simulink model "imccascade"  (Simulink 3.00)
settings: Solver=ode45  SolverMode=SingleTasking  StartTime=0.0  StopTime=100  FixedStep=st_size  MaxStep=st_size  RelTol=1e-5  AbsTol=1e-6
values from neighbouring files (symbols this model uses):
  Disturb = Setpoint    [mimo_MSF1DF_sim.m]    (also in mimo_MSF2DF_sim.m)
  Satlb = temp1    [cback.m]    (also in imcmenu.m = str2num(satlbs))
  Satub = temp1    [cback.m]    (also in imcmenu.m = str2num(satubs))
  Setpoint = zeros(1,n)    [mimo_MSF1DF_sim.m]    (also in mimo_MSF2DF_sim.m)
undefined symbols (not defined in the file or in its folder): denCs, denCs2, numCs, numCs2, Qdden, Qdnum, XdenMs, XdenPs, Xmdeadx, XnumMs, XnumPs, Xpdeadx

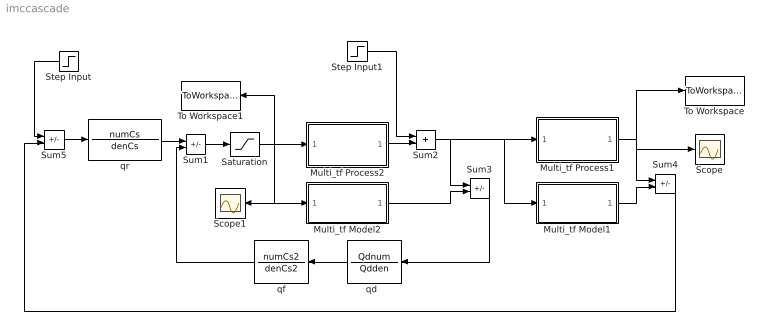
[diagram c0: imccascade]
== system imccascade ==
  Multi_tf Model1 : Subsystem
  Multi_tf Model2 : Subsystem
  Multi_tf Process1 : Subsystem
  Multi_tf Process2 : Subsystem
  Saturation : Saturate  UpperLimit=Satub  LowerLimit=Satlb
  Scope : Scope
  Scope1 : Scope
  Step Input : Step  Orientation=left  Time=0  Before=0  After=Setpoint  SampleTime=0
  Step Input1 : Step  Time=0  Before=0  After=Disturb  SampleTime=0
  Sum{1,3..5} (4 alike) : Sum  Inputs=+-  SaturateOnIntegerOverflow=on
  Sum2 : Sum  Inputs=++  SaturateOnIntegerOverflow=on
  To Workspace : ToWorkspace  VariableName=simout  SampleTime=-1  SaveFormat=Matrix
  To Workspace1 : ToWorkspace  VariableName=effort  SampleTime=-1  SaveFormat=Matrix
  "qd  " : TransferFcn  Orientation=left  Numerator=Qdnum  Denominator=Qdden
  qf : TransferFcn  Orientation=left  Numerator=numCs2  Denominator=denCs2
  qr : TransferFcn  Numerator=numCs  Denominator=denCs
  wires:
  qr/1 -> Sum1/1
  Sum3/1 -> "qd  "/1
  "qd  "/1 -> qf/1
  qf/1 -> Sum1/2
  Sum1/1 -> Saturation/1
  Multi_tf Model2/1(Out1) -> Sum3/2
  Saturation/1 -> Multi_tf Process2/1(In1), Multi_tf Model2/1(In1), Scope1/1, To Workspace1/1
  Multi_tf Process2/1(Out1) -> Sum2/2
  Step Input1/1 -> Sum2/1
  Sum2/1 -> Sum3/1, Multi_tf Process1/1(In1), Multi_tf Model1/1(In1)
  Multi_tf Model1/1(Out1) -> Sum4/2
  Multi_tf Process1/1(Out1) -> To Workspace/1, Sum4/1, Scope/1
  Sum4/1 -> Sum5/2
  Sum5/1 -> qr/1
  Step Input/1 -> Sum5/1

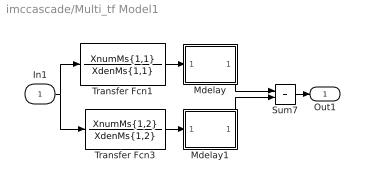
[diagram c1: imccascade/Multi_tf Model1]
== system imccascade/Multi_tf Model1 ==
  In1 : Inport  Port=1  PortWidth=-1  SampleTime=-1  DataType=auto
  Mdelay : Subsystem
  Mdelay1 : Subsystem
  Sum7 : Sum  Inputs=++  SaturateOnIntegerOverflow=on
  Transfer Fcn1 : TransferFcn  Numerator=XnumMs{1,1}  Denominator=XdenMs{1,1}
  Transfer Fcn3 : TransferFcn  Numerator=XnumMs{1,2}  Denominator=XdenMs{1,2}
  Out1 : Outport  Port=1  InitialOutput=0
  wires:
  Transfer Fcn1/1 -> Mdelay/1(In1)
  Transfer Fcn3/1 -> Mdelay1/1(In1)
  In1/1 -> Transfer Fcn1/1, Transfer Fcn3/1
  Sum7/1 -> Out1/1
  Mdelay/1(Out1) -> Sum7/1
  Mdelay1/1(Out1) -> Sum7/2

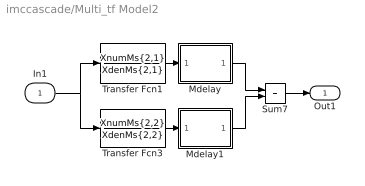
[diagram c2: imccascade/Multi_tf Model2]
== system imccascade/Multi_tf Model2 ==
  In1 : Inport  Port=1  PortWidth=-1  SampleTime=-1  DataType=auto
  Mdelay : Subsystem
  Mdelay1 : Subsystem
  Sum7 : Sum  Inputs=++  SaturateOnIntegerOverflow=on
  Transfer Fcn1 : TransferFcn  Numerator=XnumMs{2,1}  Denominator=XdenMs{2,1}
  Transfer Fcn3 : TransferFcn  Numerator=XnumMs{2,2}  Denominator=XdenMs{2,2}
  Out1 : Outport  Port=1  InitialOutput=0
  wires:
  Transfer Fcn1/1 -> Mdelay/1(In1)
  Mdelay/1(Out1) -> Sum7/1
  Mdelay1/1(Out1) -> Sum7/2
  Transfer Fcn3/1 -> Mdelay1/1(In1)
  In1/1 -> Transfer Fcn1/1, Transfer Fcn3/1
  Sum7/1 -> Out1/1

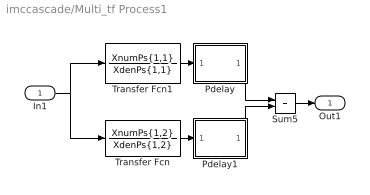
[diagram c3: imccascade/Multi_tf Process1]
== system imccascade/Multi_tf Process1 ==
  In1 : Inport  Port=1  PortWidth=-1  SampleTime=-1  DataType=auto
  Pdelay : Subsystem
  Pdelay1 : Subsystem
  Sum5 : Sum  Inputs=++  SaturateOnIntegerOverflow=on
  Transfer Fcn : TransferFcn  Numerator=XnumPs{1,2}  Denominator=XdenPs{1,2}
  Transfer Fcn1 : TransferFcn  Numerator=XnumPs{1,1}  Denominator=XdenPs{1,1}
  Out1 : Outport  Port=1  InitialOutput=0
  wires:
  Transfer Fcn1/1 -> Pdelay/1(In1)
  Transfer Fcn/1 -> Pdelay1/1(In1)
  Pdelay/1(Out1) -> Sum5/1
  In1/1 -> Transfer Fcn1/1, Transfer Fcn/1
  Sum5/1 -> Out1/1
  Pdelay1/1(Out1) -> Sum5/2

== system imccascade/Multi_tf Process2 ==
  In1 : Inport  Port=1  PortWidth=-1  SampleTime=-1  DataType=auto
  Pdelay : Subsystem
  Pdelay1 : Subsystem
  Sum5 : Sum  Inputs=++  SaturateOnIntegerOverflow=on
  Transfer Fcn : TransferFcn  Numerator=XnumPs{2,2}  Denominator=XdenPs{2,2}
  Transfer Fcn1 : TransferFcn  Numerator=XnumPs{2,1}  Denominator=XdenPs{2,1}
  Out1 : Outport  Port=1  InitialOutput=0
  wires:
  Transfer Fcn1/1 -> Pdelay/1(In1)
  Transfer Fcn/1 -> Pdelay1/1(In1)
  Pdelay/1(Out1) -> Sum5/1
  Pdelay1/1(Out1) -> Sum5/2
  In1/1 -> Transfer Fcn1/1, Transfer Fcn/1
  Sum5/1 -> Out1/1

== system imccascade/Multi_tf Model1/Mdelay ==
  In1 : Inport  Port=1  PortWidth=-1  SampleTime=-1  DataType=auto
  Mdelay > 0 : TransportDelay  DelayTime=Xmdeadx{1,1}  InitialInput=0  BufferSize=1024
  Mdelay = 0 : Subsystem  Description=pass input signal through out1 if condition is true.
  Sum6 : Sum  Inputs=++  SaturateOnIntegerOverflow=on
  Out1 : Outport  Port=1
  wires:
  Mdelay = 0/1(Out2) -> Mdelay > 0/1
  Mdelay > 0/1 -> Sum6/1
  Mdelay = 0/2(Out1) -> Sum6/2
  In1/1 -> Mdelay = 0/1(In)
  Sum6/1 -> Out1/1

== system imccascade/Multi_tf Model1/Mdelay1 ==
  In1 : Inport  Port=1  PortWidth=-1  SampleTime=-1  DataType=auto
  Mdelay > 0 : TransportDelay  DelayTime=Xmdeadx{1,2}  InitialInput=0  BufferSize=1024
  Mdelay = 0 : Subsystem  Description=pass input signal through out1 if condition is true.
  Sum6 : Sum  Inputs=++  SaturateOnIntegerOverflow=on
  Out1 : Outport  Port=1
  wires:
  Mdelay = 0/1(Out2) -> Mdelay > 0/1
  Mdelay > 0/1 -> Sum6/1
  Mdelay = 0/2(Out1) -> Sum6/2
  In1/1 -> Mdelay = 0/1(In)
  Sum6/1 -> Out1/1

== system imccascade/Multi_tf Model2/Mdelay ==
  In1 : Inport  Port=1  PortWidth=-1  SampleTime=-1  DataType=auto
  Mdelay > 0 : TransportDelay  DelayTime=Xmdeadx{2,1}  InitialInput=0  BufferSize=1024
  Mdelay = 0 : Subsystem  Description=pass input signal through out1 if condition is true.
  Sum6 : Sum  Inputs=++  SaturateOnIntegerOverflow=on
  Out1 : Outport  Port=1
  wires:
  Mdelay = 0/1(Out2) -> Mdelay > 0/1
  Mdelay > 0/1 -> Sum6/1
  Mdelay = 0/2(Out1) -> Sum6/2
  In1/1 -> Mdelay = 0/1(In)
  Sum6/1 -> Out1/1

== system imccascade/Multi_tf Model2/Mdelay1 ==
  In1 : Inport  Port=1  PortWidth=-1  SampleTime=-1  DataType=auto
  Mdelay > 0 : TransportDelay  DelayTime=Xmdeadx{2,2}  InitialInput=0  BufferSize=1024
  Mdelay = 0 : Subsystem  Description=pass input signal through out1 if condition is true.
  Sum6 : Sum  Inputs=++  SaturateOnIntegerOverflow=on
  Out1 : Outport  Port=1
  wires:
  Mdelay = 0/1(Out2) -> Mdelay > 0/1
  Mdelay > 0/1 -> Sum6/1
  Mdelay = 0/2(Out1) -> Sum6/2
  In1/1 -> Mdelay = 0/1(In)
  Sum6/1 -> Out1/1

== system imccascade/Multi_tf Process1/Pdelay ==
  In1 : Inport  Port=1  PortWidth=-1  SampleTime=-1  DataType=auto
  Mdelay > 0 : TransportDelay  DelayTime=Xpdeadx{1,1}  InitialInput=0  BufferSize=1024
  Mdelay = 0 : Subsystem  Description=pass input signal through out1 if condition is true.
  Sum6 : Sum  Inputs=++  SaturateOnIntegerOverflow=on
  Out1 : Outport  Port=1
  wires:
  Mdelay = 0/1(Out2) -> Mdelay > 0/1
  Mdelay > 0/1 -> Sum6/1
  Mdelay = 0/2(Out1) -> Sum6/2
  In1/1 -> Mdelay = 0/1(In)
  Sum6/1 -> Out1/1

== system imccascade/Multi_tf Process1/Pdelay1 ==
  In1 : Inport  Port=1  PortWidth=-1  SampleTime=-1  DataType=auto
  Mdelay > 0 : TransportDelay  DelayTime=Xpdeadx{1,2}  InitialInput=0  BufferSize=1024
  Mdelay = 0 : Subsystem  Description=pass input signal through out1 if condition is true.
  Sum6 : Sum  Inputs=++  SaturateOnIntegerOverflow=on
  Out1 : Outport  Port=1
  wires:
  Mdelay = 0/1(Out2) -> Mdelay > 0/1
  Mdelay > 0/1 -> Sum6/1
  Mdelay = 0/2(Out1) -> Sum6/2
  In1/1 -> Mdelay = 0/1(In)
  Sum6/1 -> Out1/1

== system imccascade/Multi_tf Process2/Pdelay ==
  In1 : Inport  Port=1  PortWidth=-1  SampleTime=-1  DataType=auto
  Mdelay > 0 : TransportDelay  DelayTime=Xpdeadx{2,1}  InitialInput=0  BufferSize=1024
  Mdelay = 0 : Subsystem  Description=pass input signal through out1 if condition is true.
  Sum6 : Sum  Inputs=++  SaturateOnIntegerOverflow=on
  Out1 : Outport  Port=1
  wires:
  Mdelay = 0/1(Out2) -> Mdelay > 0/1
  Mdelay > 0/1 -> Sum6/1
  Mdelay = 0/2(Out1) -> Sum6/2
  In1/1 -> Mdelay = 0/1(In)
  Sum6/1 -> Out1/1

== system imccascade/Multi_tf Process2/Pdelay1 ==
  In1 : Inport  Port=1  PortWidth=-1  SampleTime=-1  DataType=auto
  Mdelay > 0 : TransportDelay  DelayTime=Xpdeadx{2,2}  InitialInput=0  BufferSize=1024
  Mdelay = 0 : Subsystem  Description=pass input signal through out1 if condition is true.
  Sum6 : Sum  Inputs=++  SaturateOnIntegerOverflow=on
  Out1 : Outport  Port=1
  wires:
  Mdelay = 0/1(Out2) -> Mdelay > 0/1
  Mdelay > 0/1 -> Sum6/1
  Mdelay = 0/2(Out1) -> Sum6/2
  In1/1 -> Mdelay = 0/1(In)
  Sum6/1 -> Out1/1

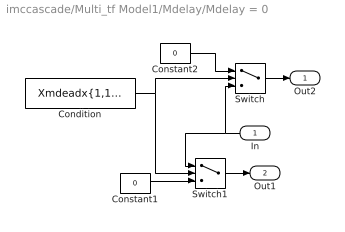
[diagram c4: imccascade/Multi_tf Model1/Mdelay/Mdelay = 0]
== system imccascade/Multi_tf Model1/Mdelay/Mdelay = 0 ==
  In : Inport  Orientation=left  Port=1  PortWidth=-1  SampleTime=-1  DataType=auto
  Condition : Constant  Value=Xmdeadx{1,1}<=3*eps
  Constant1 : Constant  Value=0
  Constant2 : Constant  Value=0
  Switch : Switch  Threshold=1
  Switch1 : Switch  Threshold=1
  Out2 : Outport  Port=1  InitialOutput=0
  Out1 : Outport  Port=2  InitialOutput=0
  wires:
  In/1 -> Switch/3, Switch1/1
  Condition/1 -> Switch1/2, Switch/2
  Constant1/1 -> Switch1/3
  Constant2/1 -> Switch/1
  Switch/1 -> Out2/1
  Switch1/1 -> Out1/1

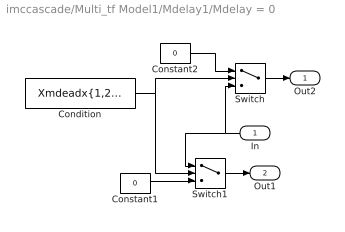
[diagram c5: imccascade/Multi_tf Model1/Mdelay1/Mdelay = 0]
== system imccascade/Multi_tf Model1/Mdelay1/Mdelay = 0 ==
  In : Inport  Orientation=left  Port=1  PortWidth=-1  SampleTime=-1  DataType=auto
  Condition : Constant  Value=Xmdeadx{1,2}<=3*eps
  Constant1 : Constant  Value=0
  Constant2 : Constant  Value=0
  Switch : Switch  Threshold=1
  Switch1 : Switch  Threshold=1
  Out2 : Outport  Port=1  InitialOutput=0
  Out1 : Outport  Port=2  InitialOutput=0
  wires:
  In/1 -> Switch/3, Switch1/1
  Condition/1 -> Switch1/2, Switch/2
  Constant1/1 -> Switch1/3
  Constant2/1 -> Switch/1
  Switch/1 -> Out2/1
  Switch1/1 -> Out1/1

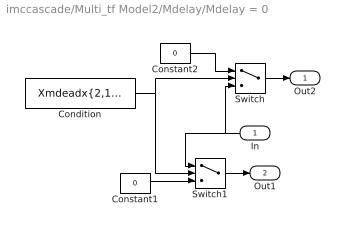
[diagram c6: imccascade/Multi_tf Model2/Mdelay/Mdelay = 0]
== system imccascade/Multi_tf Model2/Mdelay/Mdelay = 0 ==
  In : Inport  Orientation=left  Port=1  PortWidth=-1  SampleTime=-1  DataType=auto
  Condition : Constant  Value=Xmdeadx{2,1}<=3*eps
  Constant1 : Constant  Value=0
  Constant2 : Constant  Value=0
  Switch : Switch  Threshold=1
  Switch1 : Switch  Threshold=1
  Out2 : Outport  Port=1  InitialOutput=0
  Out1 : Outport  Port=2  InitialOutput=0
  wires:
  In/1 -> Switch/3, Switch1/1
  Condition/1 -> Switch1/2, Switch/2
  Constant1/1 -> Switch1/3
  Constant2/1 -> Switch/1
  Switch/1 -> Out2/1
  Switch1/1 -> Out1/1

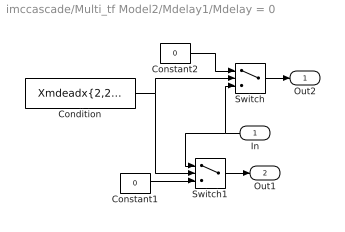
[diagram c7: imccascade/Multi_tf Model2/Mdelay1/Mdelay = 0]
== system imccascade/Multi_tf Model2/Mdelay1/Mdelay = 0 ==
  In : Inport  Orientation=left  Port=1  PortWidth=-1  SampleTime=-1  DataType=auto
  Condition : Constant  Value=Xmdeadx{2,2}<=3*eps
  Constant1 : Constant  Value=0
  Constant2 : Constant  Value=0
  Switch : Switch  Threshold=1
  Switch1 : Switch  Threshold=1
  Out2 : Outport  Port=1  InitialOutput=0
  Out1 : Outport  Port=2  InitialOutput=0
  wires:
  In/1 -> Switch/3, Switch1/1
  Condition/1 -> Switch1/2, Switch/2
  Constant1/1 -> Switch1/3
  Constant2/1 -> Switch/1
  Switch/1 -> Out2/1
  Switch1/1 -> Out1/1

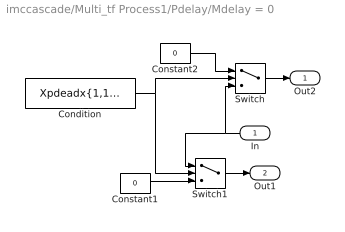
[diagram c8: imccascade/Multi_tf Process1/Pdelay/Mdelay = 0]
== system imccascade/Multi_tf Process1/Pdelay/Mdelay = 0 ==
  In : Inport  Orientation=left  Port=1  PortWidth=-1  SampleTime=-1  DataType=auto
  Condition : Constant  Value=Xpdeadx{1,1}<=3*eps
  Constant1 : Constant  Value=0
  Constant2 : Constant  Value=0
  Switch : Switch  Threshold=1
  Switch1 : Switch  Threshold=1
  Out2 : Outport  Port=1  InitialOutput=0
  Out1 : Outport  Port=2  InitialOutput=0
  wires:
  In/1 -> Switch/3, Switch1/1
  Condition/1 -> Switch1/2, Switch/2
  Constant1/1 -> Switch1/3
  Constant2/1 -> Switch/1
  Switch/1 -> Out2/1
  Switch1/1 -> Out1/1

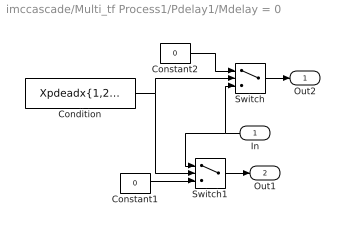
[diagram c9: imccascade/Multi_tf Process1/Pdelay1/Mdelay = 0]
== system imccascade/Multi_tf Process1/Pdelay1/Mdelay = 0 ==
  In : Inport  Orientation=left  Port=1  PortWidth=-1  SampleTime=-1  DataType=auto
  Condition : Constant  Value=Xpdeadx{1,2}<=3*eps
  Constant1 : Constant  Value=0
  Constant2 : Constant  Value=0
  Switch : Switch  Threshold=1
  Switch1 : Switch  Threshold=1
  Out2 : Outport  Port=1  InitialOutput=0
  Out1 : Outport  Port=2  InitialOutput=0
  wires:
  In/1 -> Switch/3, Switch1/1
  Condition/1 -> Switch1/2, Switch/2
  Constant1/1 -> Switch1/3
  Constant2/1 -> Switch/1
  Switch/1 -> Out2/1
  Switch1/1 -> Out1/1

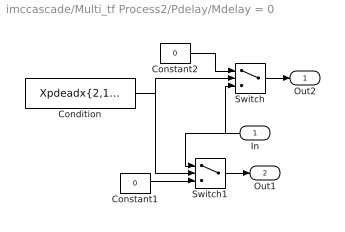
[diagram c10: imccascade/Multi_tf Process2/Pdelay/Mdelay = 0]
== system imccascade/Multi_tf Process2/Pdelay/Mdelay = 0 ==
  In : Inport  Orientation=left  Port=1  PortWidth=-1  SampleTime=-1  DataType=auto
  Condition : Constant  Value=Xpdeadx{2,1}<=3*eps
  Constant1 : Constant  Value=0
  Constant2 : Constant  Value=0
  Switch : Switch  Threshold=1
  Switch1 : Switch  Threshold=1
  Out2 : Outport  Port=1  InitialOutput=0
  Out1 : Outport  Port=2  InitialOutput=0
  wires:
  In/1 -> Switch/3, Switch1/1
  Condition/1 -> Switch1/2, Switch/2
  Constant1/1 -> Switch1/3
  Constant2/1 -> Switch/1
  Switch/1 -> Out2/1
  Switch1/1 -> Out1/1

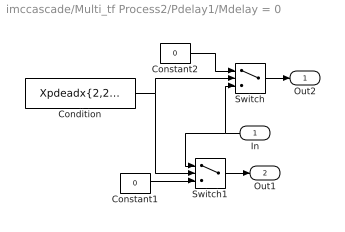
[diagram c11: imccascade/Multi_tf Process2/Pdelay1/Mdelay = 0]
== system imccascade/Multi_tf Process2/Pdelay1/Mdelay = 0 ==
  In : Inport  Orientation=left  Port=1  PortWidth=-1  SampleTime=-1  DataType=auto
  Condition : Constant  Value=Xpdeadx{2,2}<=3*eps
  Constant1 : Constant  Value=0
  Constant2 : Constant  Value=0
  Switch : Switch  Threshold=1
  Switch1 : Switch  Threshold=1
  Out2 : Outport  Port=1  InitialOutput=0
  Out1 : Outport  Port=2  InitialOutput=0
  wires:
  In/1 -> Switch/3, Switch1/1
  Condition/1 -> Switch1/2, Switch/2
  Constant1/1 -> Switch1/3
  Constant2/1 -> Switch/1
  Switch/1 -> Out2/1
  Switch1/1 -> Out1/1
